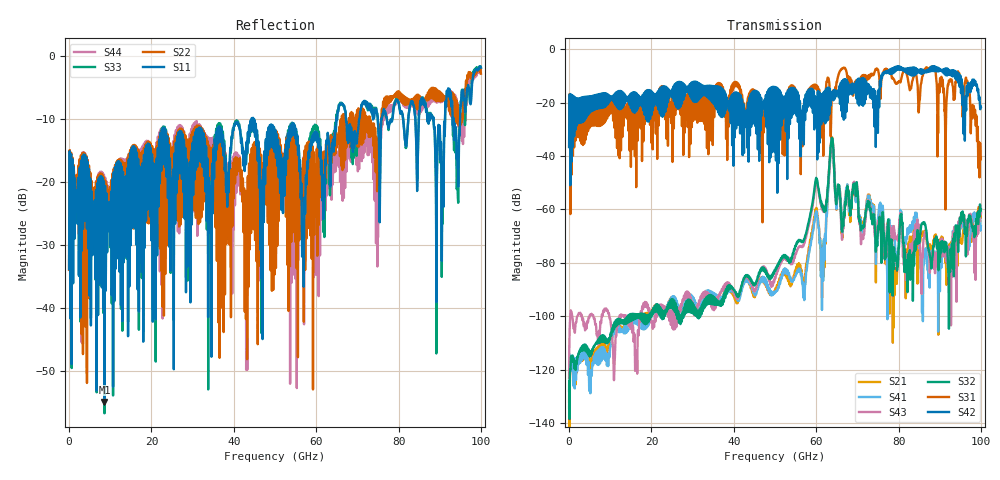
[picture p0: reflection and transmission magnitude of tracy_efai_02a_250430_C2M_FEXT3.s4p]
!! PART DESCRIPTION: TE 224G+ VSR Channel- Chip to module, IO connector to CPC(Co-packaged connector) through over the board cable
!! CHANNEL DESCRIPTION: Module trace -> Mated IO 224G+ Connector -> Internal Cable Termination -> 30AWG 300mm Cable -> Cable
!!  termination + CPC connector(No footprint or package included)
!! MODEL REVISION:  Rev 3, Created on April 29, 2025
!! MODEL STATUS: Development
!! MODEL GEOMETRY: FEXT3
!! MODEL FREQUENCY RANGE: 0 GHz to 100 GHz in 10.00 MHz frequency steps
!! PORT DEFINITIONS:
!! Port  1  ----->  Module Side  -->  Host Side  <-----  Port  2
!! Port  3  ----->  Module Side  -->  Host Side  <-----  Port  4
# HZ S MA R 45.000000
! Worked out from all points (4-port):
!   10000 points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, 10 MHz to 100 GHz, reference 45 ohm
!   strongest paths, dB at 10 MHz, 25.01 GHz, 50.01 GHz, 75.01 GHz, 100 GHz:
!     S42: -36.7, -15.5, -15.5, -28.4, -21.6
!     S31: -36.5, -17.8, -16.0, -7.7, -40.6
!     S32: -128.0, -97.0, -83.1, -67.1, -59.9
!     S43: -123.1, -102.6, -85.7, -64.6, -61.4
!     S41: -134.2, -95.6, -90.8, -63.4, -66.3
!     S21: -132.0, -95.6, -90.5, -64.5, -61.1
!   lowest |S11| = -54.9 dB at 8.6 GHz (marker M1), VSWR 1.00, Z = 44.9 + j0.15 ohm
!   |S11| at or under -10 dB: start of sweep to 44.32 GHz; 44.72 GHz to 64.9 GHz (20.18 GHz wide, 36.8 % of centre); 67.23 GHz to 70.41 GHz (3.185 GHz wide, 4.63 % of centre)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
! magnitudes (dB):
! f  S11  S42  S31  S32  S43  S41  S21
! 10 MHz  -33.8  -36.7  -36.5  -128.0  -123.1  -134.2  -132.0
! 8.6 GHz  -54.9  -21.6  -27.5  -108.5  -97.2  -113.2  -112.1
! 61.57 GHz  -19.4  -26.7  -26.8  -58.6  -59.4  -74.6  -74.0
! 63.82 GHz  -13.9  -17.5  -17.3  -33.2  -34.4  -34.0  -32.9
! 79.03 GHz  -7.6  -8.4  -12.1  -79.1  -68.4  -69.2  -91.9
! 94.55 GHz  -18.1  -11.6  -9.1  -68.4  -64.7  -64.8  -69.6
! 100 GHz  -1.8  -21.6  -40.6  -59.9  -61.4  -66.3  -61.1
